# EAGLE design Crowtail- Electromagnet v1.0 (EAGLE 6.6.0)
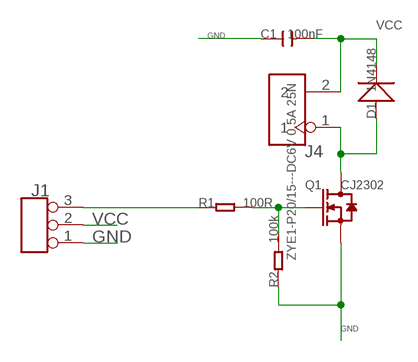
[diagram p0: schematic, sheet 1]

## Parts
C1  100nF  C-0603  [C0603]
D1  1N4148  D'1N4148-SMD'  [LL-34]
J1  TINKER_3P_DIP  [3P_2.0_DIP]
J4  ZYE1-P20/15---DC6V 0.5A 25N  HEADER-2P-65/35MIL  [2P-2.54-65/35MIL]
Q1  CJ2302  MOSFET-N'SOT23'  [SOT23]
R1  100R  R-0603  [R0603]
R2  100k  R-0603  [R0603]

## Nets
GND: C1.1 J1.1 Q1.2(S) R2.1
N$1: J1.3 R1.1
N$4: Q1.1(G) R1.2 R2.2
N$7: D1.A(+) J4.1 Q1.3(D)
VCC: C1.2 D1.C(-) J1.2 J4.2

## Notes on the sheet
- GND
- GND

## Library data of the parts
C1 = Discrete:C*: Ceramic Capacitors
D1 = Discrete:D*
J1 = Connector:TINKER_3P_DIP
J4 = Connector :HEADER-2P
Q1 = Discrete:MOSFET-N: IRLL014: http://www.vishay.com/docs/91319/sihll014.pdf
R1 R2 = Discrete:R*

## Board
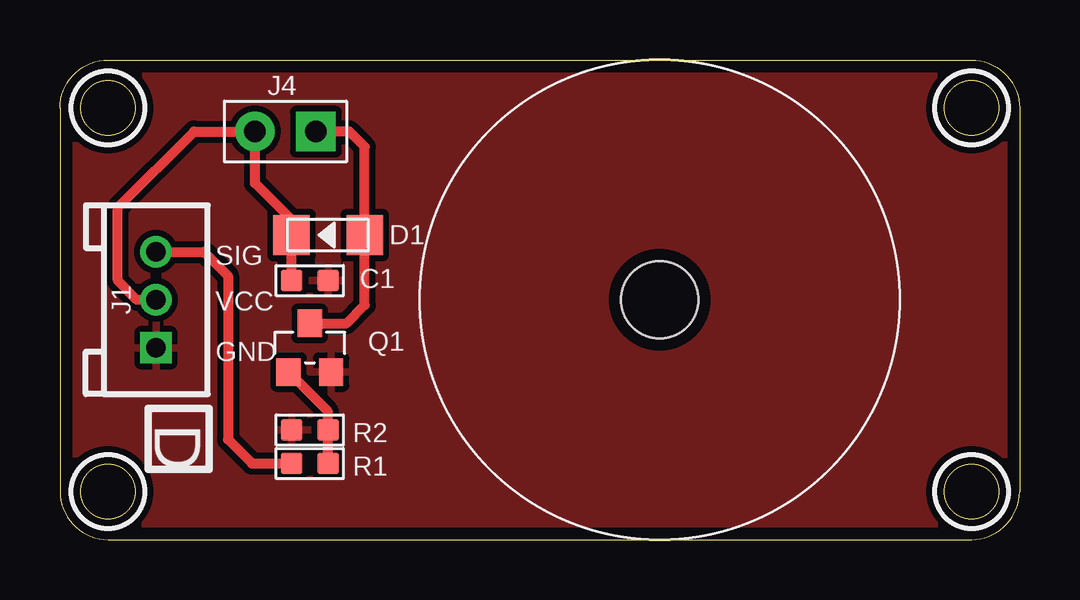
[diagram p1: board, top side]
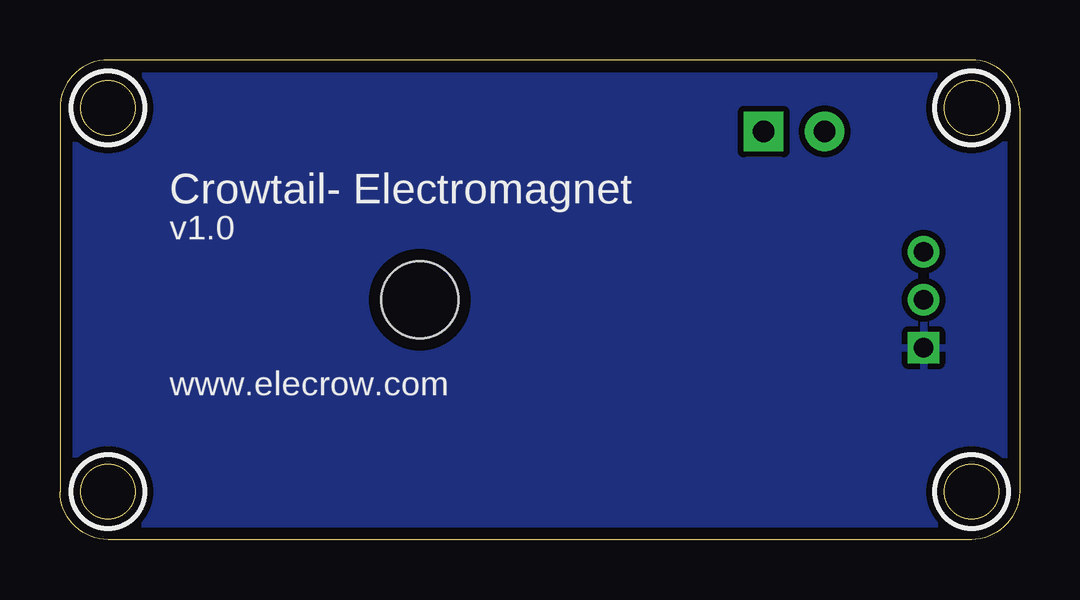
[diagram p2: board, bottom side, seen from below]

Size 40 x 20 mm. Coordinates in mm from the lower left corner, seen from the top.
Outline: 0,18 0,2 arc90 2,0 38,0 arc90 40,2 40,18 arc90 38,20 2,20 arc90 0,18
Outline: circle at 2,18 radius 1.14
Outline: circle at 2,18 radius 1.14
Outline: circle at 2,2 radius 1.14
Outline: circle at 38,18 radius 1.14
Outline: circle at 38,18 radius 1.14
Outline: circle at 38,2 radius 1.14
Outline: circle at 38,2 radius 1.14
Copper layers (1*16): Top 0.035mm / dielectric 1.5mm / Bottom 0.035mm
Design rules "default *": minimum track width 10mil, minimum drill 24mil, track to track 8mil, track to pad 8mil, pad to pad 8mil, via to via 8mil, smd to smd 8mil, copper to edge 20mil, drill to drill 8mil, minimum pad ring 10mil, minimum via ring 8mil, stop-mask expansion 4mil, vias tented up to drill 100mil, thermal gap 10mil
Holes 3.2 mm at 25,10
tRestrict: area 0.5,16.5 to 3.5,19.5; area 0.5,0.5 to 3.5,3.5; area 36.5,16.5 to 39.5,19.5; area 36.5,0.5 to 39.5,3.5
bRestrict: area 0.5,16.5 to 3.5,19.5; area 0.5,0.5 to 3.5,3.5; area 36.5,16.5 to 39.5,19.5; area 36.5,0.5 to 39.5,3.5

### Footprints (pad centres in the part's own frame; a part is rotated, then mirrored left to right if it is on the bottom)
C0603 = smd 0.889 x 0.889: 1 -0.762,0; 2 0.762,0
LL-34 = smd 1.524 x 1.676: A -1.524,0; C 1.524,0
3P_2.0_DIP = drill 0.8 pad 1.27 square: 1 -2,0 | drill 0.8 pad 1.27: 2 0,0; 3 2,0
2P-2.54-65/35MIL = drill 0.889 pad 1.651 square: 1 0,1.27 | drill 0.889 pad 1.651: 2 0,-1.27
SOT23 = smd 1.016 x 1.143: 1 -0.889,-1.016; 2 0.889,-1.016; 3 0,1.016
R0603 = smd 0.889 x 0.889: 1 -0.762,0; 2 0.762,0

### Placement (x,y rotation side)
C1  10.41,10.79 180 top
D1  11.18,12.7 180 top
J1  4,10 90 top
J4  9.4,17.02 270 top
Q1  10.41,8 0 top
R1  10.41,3.17 0 top
R2  10.41,4.57 0 top

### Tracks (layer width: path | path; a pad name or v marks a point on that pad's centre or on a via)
GND
  pour Top (isolate 0.254): -0.76,20.83 40.89,20.83 40.89,-0.64 -0.76,-0.64
  pour Bottom (isolate 0.254): -0.64,20.7 40.77,20.7 40.77,-0.51 -0.64,-0.51
N$1
  Top 0.406: J1.3 6,12 7,11 7,4.18 8,3.17 R1.1
N$4
  Top 0.406: R1.2 R2.2 11.18,5.33 Q1.1
N$7
  Top 0.406: Q1.3 11.94,9.02 12.7,9.78 D1.A 12.7,16.38 12.06,17.02 J4.1
VCC
  Top 0.406: J1.2 3.21,10 2.41,10.79 2.41,13.84 5.59,17.02 J4.2 8.13,14.86 9.65,13.34 D1.C C1.2

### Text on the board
tPlace: D
bPlace: Crowtail- Electromagnet | v1.0 | www.elecrow.com
tNames: SIG | VCC | GND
